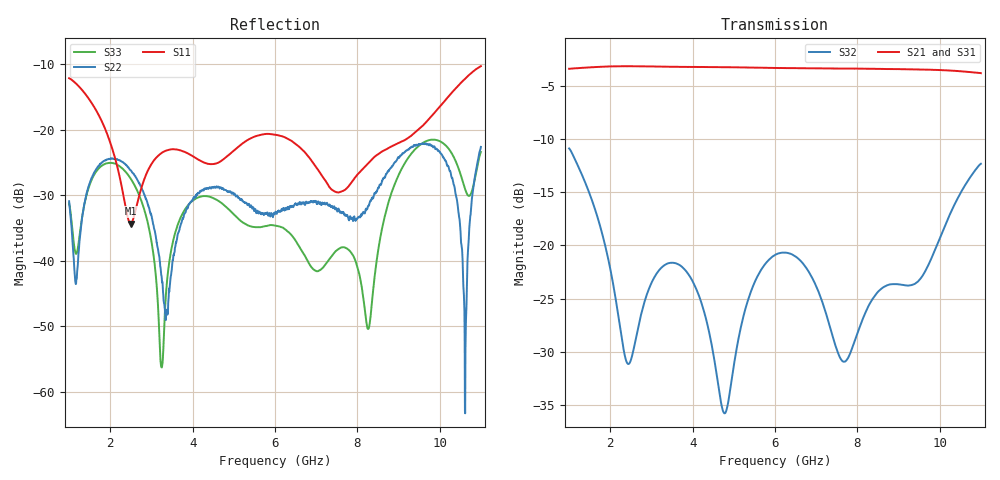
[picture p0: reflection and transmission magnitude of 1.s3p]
!The following data was pulled from an Agilent PNA
!This sNp file was generated from the data in the RF Test software
!NOTE:  Smoothing/Math/Corrections applied on any given trace ARE included in the data saved here
# MHz S dB R 50
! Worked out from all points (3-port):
!   1601 points, 1 GHz to 11 GHz, reference 50 ohm
!   strongest paths, dB at 1 GHz, 3.5 GHz, 6 GHz, 8.5 GHz, 11 GHz:
!     S21: -3.4, -3.2, -3.3, -3.4, -3.8
!     S31: -3.4, -3.3, -3.4, -3.6, -4.4
!     S32: -10.9, -21.6, -20.9, -24.4, -12.3
!   lowest |S11| = -34.3 dB at 2.494 GHz (marker M1), VSWR 1.04, Z = 48.3 + j0.914 ohm
!   |S11| at or under -10 dB: start of sweep to end of sweep
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1000  -12.16 134.0  -3.40 -64.8  -3.42 -64.0
      -3.40 -63.9  -30.93 33.1  -10.90 -86.3
      -3.43 -64.0  -10.89 -86.3  -31.25 24.1
2493.75  -34.34 150.5  -3.16 -163.5  -3.19 -163.6
         -3.16 -163.5  -26.20 115.8  -30.84 -79.6
         -3.19 -163.6  -30.85 -79.6  -27.47 119.8
3243.75  -23.58 -164.1  -3.20 146.1  -3.24 145.9
         -3.20 146.1  -42.31 84.2  -22.10 -72.0
         -3.24 145.9  -22.09 -72.0  -56.29 -24.8
3900  -23.69 -173.3  -3.22 101.9  -3.27 101.7
      -3.22 101.9  -31.49 174.5  -22.74 -107.7
      -3.26 101.7  -22.73 -107.7  -31.45 -165.2
4781.25  -24.37 -146.4  -3.25 42.0  -3.30 41.7
         -3.25 42.0  -29.21 96.9  -35.76 -85.1
         -3.31 41.7  -35.78 -85.0  -31.63 110.0
6000  -20.78 -157.7  -3.32 -41.9  -3.39 -42.3
      -3.33 -41.9  -32.88 -72.1  -20.91 -85.7
      -3.39 -42.2  -20.90 -85.6  -34.66 -70.3
7981.25  -27.02 -105.8  -3.39 178.2  -3.50 177.7
         -3.39 178.2  -33.62 118.4  -28.48 -94.0
         -3.51 177.7  -28.49 -94.1  -40.56 -28.3
9968.75  -16.73 -84.9  -3.51 31.6  -3.77 30.7
         -3.52 31.6  -23.19 25.6  -19.64 -98.4
         -3.78 30.7  -19.64 -98.4  -21.68 6.2
10612.5  -12.26 -100.1  -3.67 -17.6  -4.06 -18.6
         -3.67 -17.7  -62.95 -32.1  -14.37 -119.9
         -4.06 -18.6  -14.37 -120.0  -29.01 -84.1
11000  -10.33 -116.5  -3.81 -46.4  -4.35 -48.3
       -3.81 -47.3  -22.64 125.5  -12.33 -138.4
       -4.35 -48.3  -12.33 -138.4  -23.42 153.9
